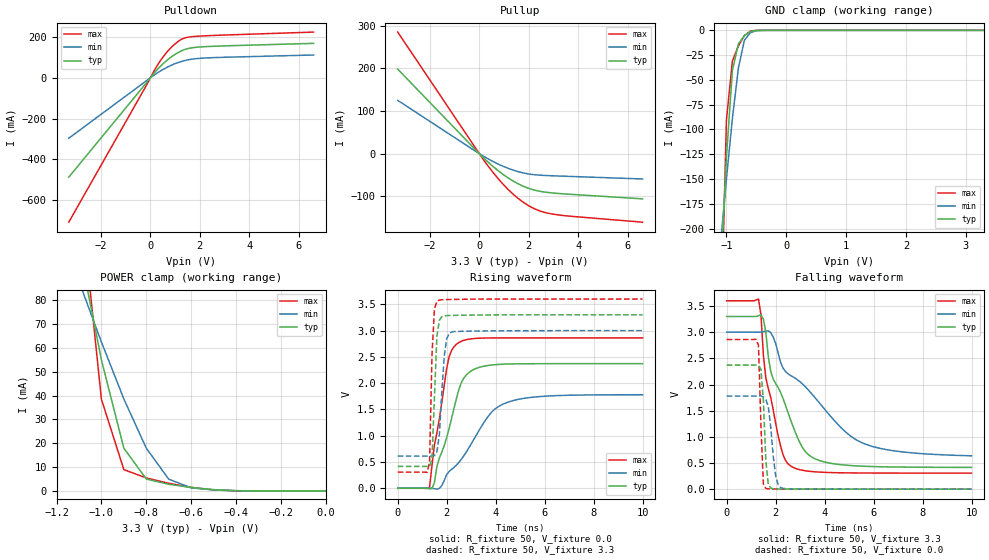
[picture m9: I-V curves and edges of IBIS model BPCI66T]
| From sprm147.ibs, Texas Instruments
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[Model]   BPCI66T
Model_type   I/O
Vinh = 2.00
Vinl = 0.80
Enable   Active-Low
Polarity   Non-Inverting
| signals   A, GZ, Y
Vmeas = 1.5
|   typ   min   max
C_comp   1.6382008p   1.6153313p   1.6672496p
|   typ   min   max
[Temperature Range]   25   -40   125
|   typ   min   max
[Voltage Range]   3.30V   3.00V   3.60V
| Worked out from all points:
|   slope of the pulldown table from 0 to 0.495 V, typ, clamps not added: 7.38 ohm
|   slope of the pullup table from 0 to 0.495 V, typ, clamps not added: 18.3 ohm
|   GND clamp passes 1 mA (typ) near -0.58 V on its own axis
|   POWER clamp passes 1 mA (typ) near -0.55 V on its own axis
|   rising waveform, R_fixture 50, V_fixture 0.0: 20-80 % time 872ps typ, 1.6ns min, 570ps max; typ from 0 V to 2.37 V
|   falling waveform, R_fixture 50, V_fixture 3.3: 20-80 % time 1.23ns typ, 2.68ns min, 680ps max; typ from 3.3 V to 0.416 V
|   rising waveform, R_fixture 50, V_fixture 3.3: 20-80 % time 149ps typ, 194ps min, 123ps max; typ from 0.416 V to 3.3 V
|   falling waveform, R_fixture 50, V_fixture 0.0: 20-80 % time 149ps typ, 236ps min, 127ps max; typ from 2.37 V to 0 V
[Pulldown]
|   Voltage   I(typ)   I(min)   I(max)
-3.3V     -488.1mA   -296.9mA   -709.5mA
-200mV    -30.51mA   -18.11mA   -45.59mA
200mV     29.53mA    17.33mA    44.51mA
600mV     78.78mA    46.93mA    116.2mA
800mV     98.59mA    59.14mA    144.1mA
1.1V      122.5mA    74.13mA    176.8mA
1.4V      139.4mA    85.1mA     196.2mA
2V        151.5mA    95.71mA    205mA
6.6V      169.3mA    112.1mA    224.7mA
[GND_clamp]
|   Voltage   I(typ)   I(min)   I(max)
-3.3V     -3.565A    -1.837A    -8.213A
-1.1V     -252.3mA   -216.4mA   -326.5mA
-1V       -128.2mA   -150.2mA   -90.65mA
-900mV    -40.45mA   -88.83mA   -30.93mA
-800mV    -13.79mA   -38.12mA   -15.74mA
-700mV    -5.362mA   -10.08mA   -5.284mA
-600mV    -1.177mA   -2.353mA   -753.1uA
-500mV    -120.9uA   -429.1uA   -44.77uA
-400mV    -7.597uA   -54.4uA    -1.355uA
3.3V      355.3pA    12.38uA    0A
[Pullup]
|   Voltage   I(typ)   I(min)   I(max)
-3.3V     198.5mA    125.1mA    285.4mA
300mV     -16.93mA   -10.42mA   -24.77mA
700mV     -37.12mA   -22.68mA   -54.5mA
1V        -50.38mA   -30.57mA   -74.2mA
1.6V      -71.63mA   -42.67mA   -106.5mA
2.2V      -85.18mA   -49.32mA   -128.6mA
2.5V      -88.91mA   -50.69mA   -135.6mA
2.9V      -91.92mA   -51.85mA   -141.2mA
3.7V      -95.5mA    -53.54mA   -147mA
6.6V      -106.2mA   -59.44mA   -160.9mA
[POWER_clamp]
|   Voltage   I(typ)   I(min)   I(max)
-3.3V     1.336A     704mA      2.888A
-1.1V     102.7mA    87.97mA    129.7mA
-1V       54.98mA    62.52mA    38.49mA
-900mV    17.93mA    38.6mA     8.936mA
-800mV    5.001mA    17.94mA    5.448mA
-700mV    2.777mA    4.928mA    3.206mA
-600mV    1.457mA    1.282mA    1.493mA
-500mV    536.1uA    428.3uA    411.4uA
-400mV    94.05uA    95.48uA    39.25uA
0V        1pA        1pA        1pA
[Ramp]
|   I(typ)   I(min)   I(max)
dV/dt_r   1.422/0.878n   1.068/1.594n   1.716/0.578n
dV/dt_f   1.730/1.229n   1.417/2.679n   1.976/0.681n
[Rising Waveform]
R_fixture = 50
V_fixture = 0.0
|  pu_on
|  TIME   V(typ)   V(min)   V(max)
0s        8nV        102nV      0V
1.3ns     -9.502mV   436.1uV    16.05mV
1.5ns     110.1mV    -8.416mV   825.2mV
2ns       965.3mV    261.2mV    2.278V
2.2ns     1.327V     358.5mV    2.622V
2.5ns     1.883V     494.3mV    2.774V
3.1ns     2.258V     922.7mV    2.848V
3.8ns     2.343V     1.43V      2.86V
4.5ns     2.364V     1.638V     2.861V
10ns      2.371V     1.779V     2.861V
[Falling Waveform]
R_fixture = 50
V_fixture = 3.3
V_fixture_min = 3.0
V_fixture_max = 3.6
|  pd_on
|  TIME   V(typ)   V(min)   V(max)
0s        3.3V       3V         3.6V
1.3ns     3.313V     3V         3.633V
1.4ns     3.334V     3.004V     3.331V
1.6ns     2.992V     3.019V     2.122V
1.8ns     2.25V      2.992V     1.749V
2.3ns     1.735V     2.316V     662.2mV
2.6ns     1.338V     2.175V     447.7mV
3.4ns     637mV      1.862V     340.5mV
5.5ns     440.4mV    893.2mV    309.1mV
10ns      416.4mV    637.8mV    307mV
[Rising Waveform]
R_fixture = 50
V_fixture = 3.3
V_fixture_min = 3.0
V_fixture_max = 3.6
|  pd_off
|  TIME   V(typ)   V(min)   V(max)
0s        415.6mV    612.6mV    307mV
1.3ns     414.9mV    613.1mV    491.1mV
1.4ns     556.3mV    611.4mV    2.539V
1.5ns     1.734V     619.7mV    3.414V
1.6ns     2.888V     695.8mV    3.558V
1.7ns     3.195V     1.018V     3.581V
1.9ns     3.28V      2.513V     3.589V
2ns       3.285V     2.844V     3.591V
2.2ns     3.289V     2.972V     3.592V
10ns      3.3V       3V         3.6V
[Falling Waveform]
R_fixture = 50
V_fixture = 0.0
|  pu_off
|  TIME   V(typ)   V(min)   V(max)
0s        2.371V     1.78V      2.861V
1.2ns     2.372V     1.78V      2.865V
1.3ns     2.367V     1.781V     2.748V
1.4ns     2.289V     1.781V     1.2V
1.5ns     1.682V     1.763V     95.66mV
1.6ns     536.5mV    1.713V     13.47mV
1.7ns     86.74mV    1.578V     6.339mV
2ns       5.603mV    259.2mV    3.472mV
2.2ns     4.231mV    30.99mV    2.284mV
10ns      11.06uV    168.1uV    1.139uV
